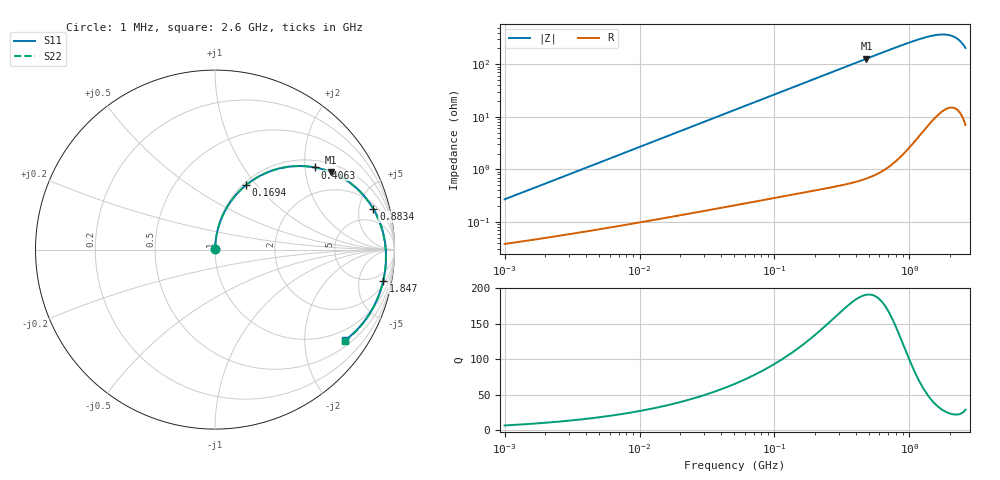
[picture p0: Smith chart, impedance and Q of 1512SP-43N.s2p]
# MHz  S  MA  R  50
!Freq  MagS11  AngS11  MagS21  AngS21  MagS12  AngS12  MagS22  AngS22
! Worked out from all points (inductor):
!   801 points, 1 MHz to 2.6 GHz, reference 50 ohm
!   read as one part in series: L = 42.5 nH near 1.04 MHz
!   highest Q = 191 at 480.2 MHz (marker M1), where L = 42.4 nH
!   S11 on the Smith chart (normalised r, x): 1 MHz: 1.00, +0.01; 169.4 MHz: 1.03, +0.89; 406.3 MHz: 1.18, +2.26; 883.4 MHz: 2.61, +6.96; 1.847 GHz: 3, -10; 2.6 GHz: 0.66, -3.05
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1  0.00261 81.4  0.9996 -0.2  0.9996 -0.2  0.00261 81.4
3.733785  0.009658 85.6  0.9993 -0.6  0.9993 -0.6  0.009657 85.6
13.80476  0.03561 86.0  0.9982 -2.2  0.9982 -2.2  0.0356 86.0
28.29582  0.07279 84.3  0.9958 -4.5  0.9958 -4.5  0.07278 84.3
51.03975  0.1304 81.1  0.9894 -8.0  0.9894 -8.0  0.1304 81.1
101.5763  0.2531 73.7  0.9647 -15.7  0.9647 -15.7  0.253 73.7
132.4574  0.3228 69.3  0.9434 -20.2  0.9434 -20.2  0.3226 69.3
169.3638  0.3996 64.3  0.9134 -25.3  0.9134 -25.3  0.3994 64.3
190.5715  0.4403 61.5  0.8945 -28.0  0.8945 -28.0  0.44 61.5
287.9972  0.595 50.2  0.8001 -39.4  0.8001 -39.4  0.5946 50.2
406.2846  0.7217 39.3  0.6884 -50.3  0.6884 -50.3  0.7212 39.3
480.1937  0.7761 33.9  0.6268 -55.8  0.6268 -55.8  0.7755 33.9
704.5917  0.8731 21.5  0.4828 -68.2  0.4828 -68.2  0.8723 21.5
883.3692  0.9112 14.4  0.4052 -75.1  0.4052 -75.1  0.9103 14.4
1075.32  0.934 8.3  0.3467 -81.0  0.3467 -81.0  0.9331 8.3
1308.98  0.9485 2.2  0.2996 -86.8  0.2996 -86.8  0.9476 2.2
1593.414  0.9549 -4.6  0.2686 -92.8  0.2686 -92.8  0.9542 -4.6
1846.61  0.9536 -10.4  0.262 -98.1  0.262 -98.1  0.9531 -10.4
2037.384  0.9482 -15.2  0.2712 -102.5  0.2712 -102.5  0.9481 -15.2
2204.098  0.9393 -19.8  0.2914 -107.0  0.2914 -107.0  0.9396 -19.8
2384.455  0.9225 -25.7  0.3307 -112.8  0.3307 -112.8  0.9235 -25.7
2600  0.8832 -34.9  0.4128 -122.3  0.4128 -122.3  0.8854 -34.9
